// TwinCAT 3 PLC project incrementBy1
// ProgramVersion: 3.1.4020.4
// libraries:
//   Tc2_Standard, * (Beckhoff Automation GmbH)
//   Tc2_System, * (Beckhoff Automation GmbH)
//   Tc3_Module, * (Beckhoff Automation GmbH)
// project tree:
//   DUTs/ ST_test.TcDUT
//   / PlcTask.TcTTO
//   POUs/ MAIN.TcPOU
// real-time tasks:
//   TASK PlcTask: cycle T#10ms, priority 20, ADS port 350

CONFIGURATION incrementBy1
    RESOURCE PLC ON TwinCAT3
        TASK PlcTask(INTERVAL := T#10ms, PRIORITY := 20);
        PROGRAM MAIN WITH PlcTask : MAIN;
    END_RESOURCE
END_CONFIGURATION

// ---- DUTs/ST_test.TcDUT
TYPE ST_test :
STRUCT
	a		:INT;
	b		:INT;
	c		:INT;
END_STRUCT
END_TYPE

// ---- POUs/MAIN.TcPOU
PROGRAM MAIN
VAR
	{attribute 'OPC.UA.DA' := '1'}
	{attribute 'OPC.UA.DA.StructuredType' :='1'}
	structure_test	:ST_test;//结构体
	
	{attribute 'OPC.UA.DA' :='1'}
	iteration3 		:INT;//整数
	{attribute 'OPC.UA.DA' :='1'}
	iter2			:INT;//整数
	{attribute 'OPC.UA.DA' := '1'}
	i			: 	INT := 0;
END_VAR

structure_test.a		:= structure_test.a + 1;
iteration3				:= iteration3 + 1; 
iter2					:= iter2 + 2;

END_PROGRAM
